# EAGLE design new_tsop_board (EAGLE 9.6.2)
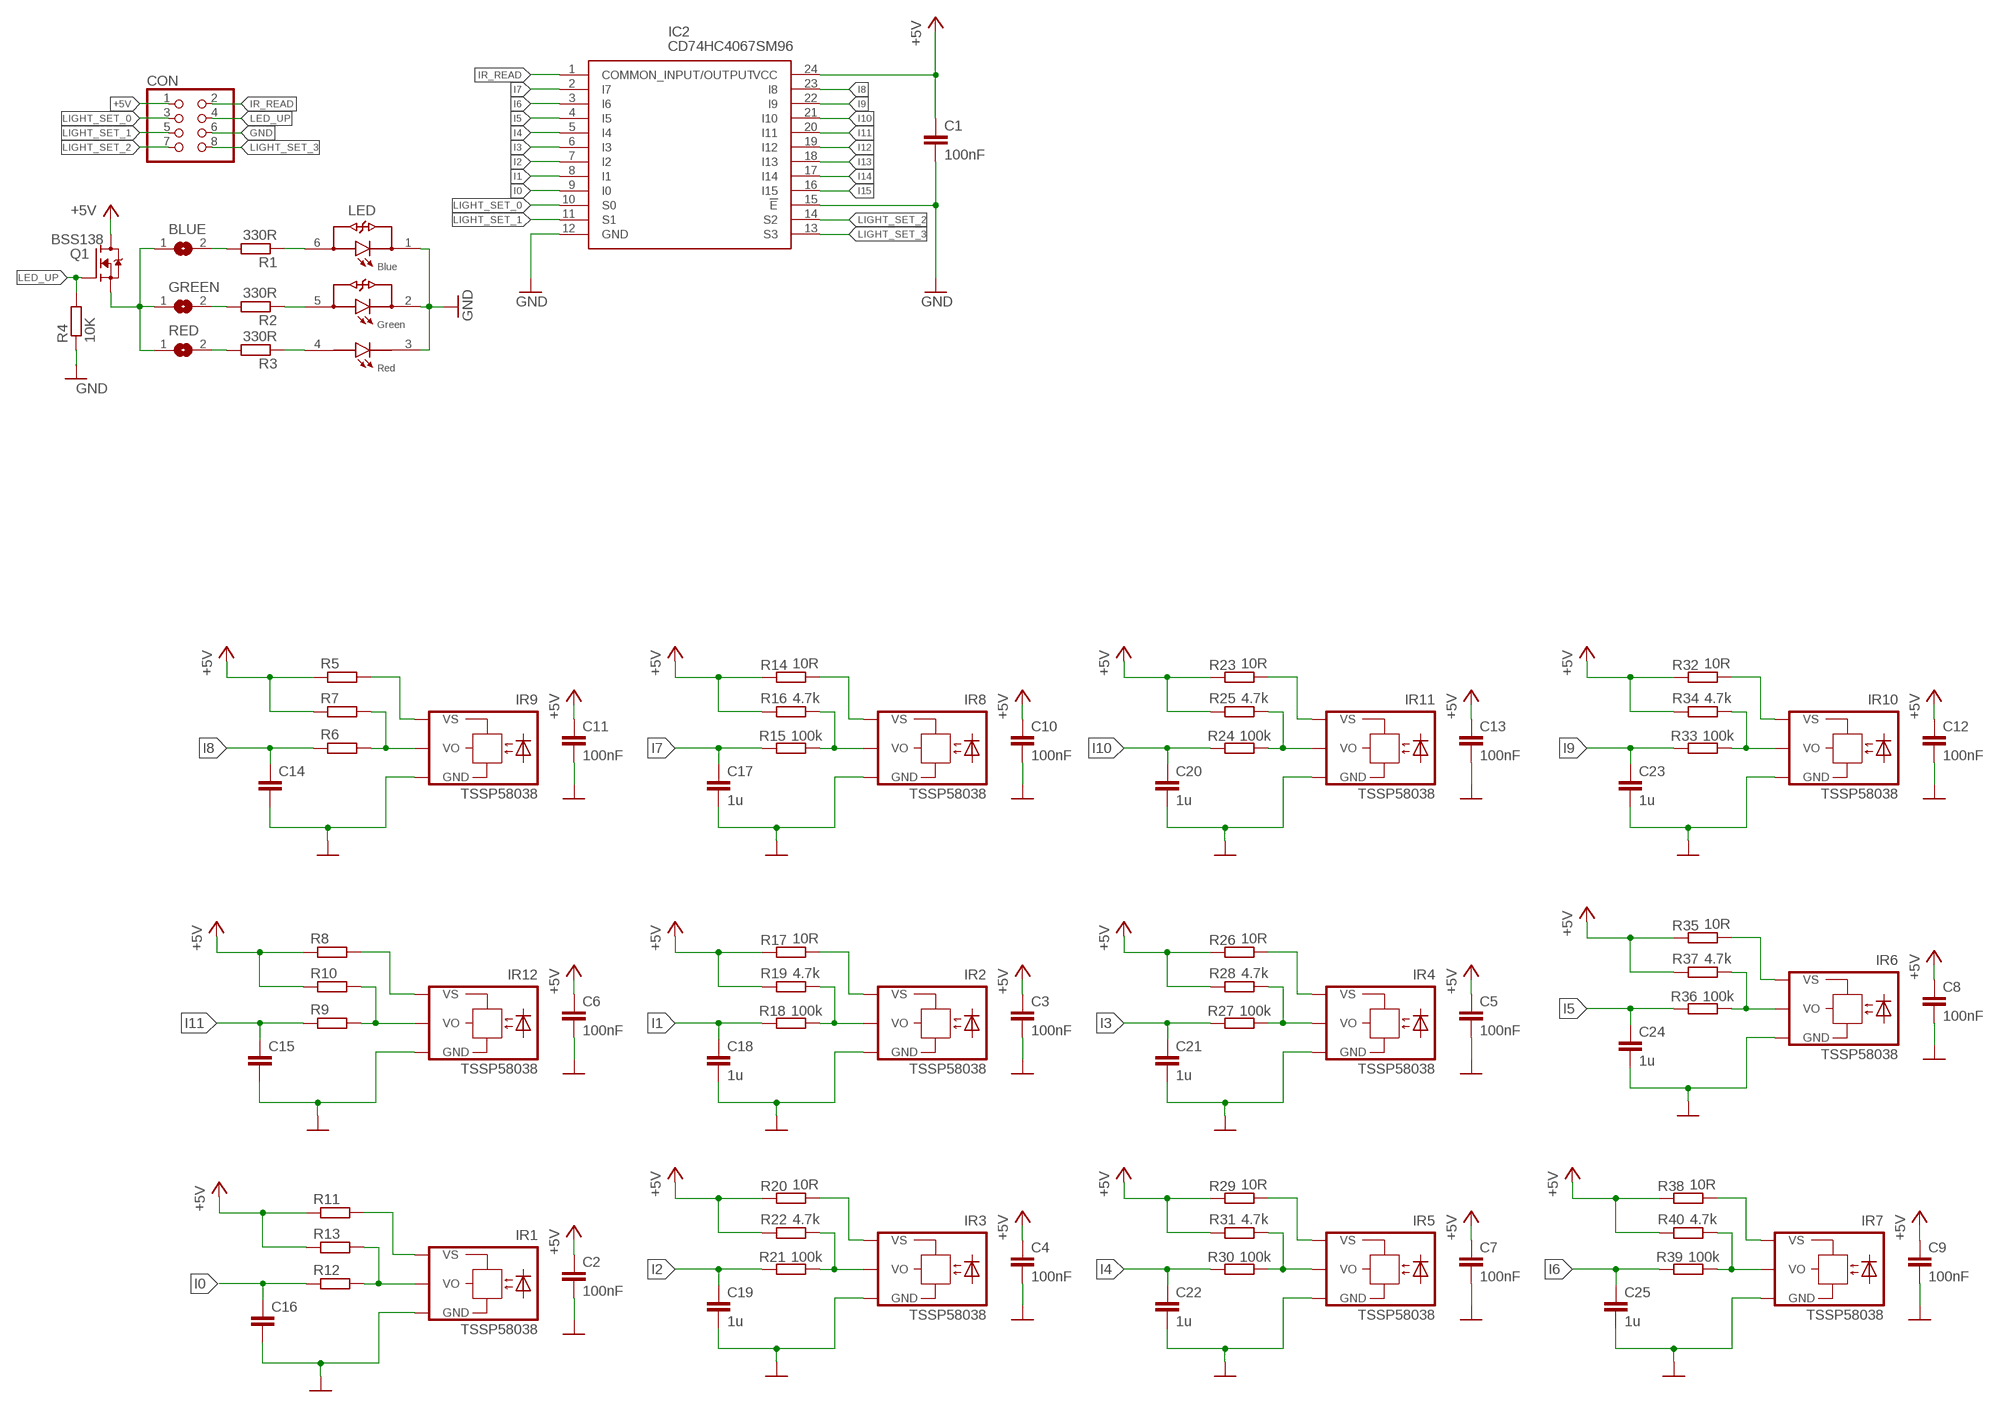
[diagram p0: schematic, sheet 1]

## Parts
BLUE  SJ  [SJ]
C1  100nF  C-EUC0805  [C0805]
C2  100nF  C-EUC0805  [C0805]
C3  100nF  C-EUC0805  [C0805]
C4  100nF  C-EUC0805  [C0805]
C5  100nF  C-EUC0805  [C0805]
C6  100nF  C-EUC0805  [C0805]
C7  100nF  C-EUC0805  [C0805]
C8  100nF  C-EUC0805  [C0805]
C9  100nF  C-EUC0805  [C0805]
C10  100nF  C-EUC0805  [C0805]
C11  100nF  C-EUC0805  [C0805]
C12  100nF  C-EUC0805  [C0805]
C13  100nF  C-EUC0805  [C0805]
C14  C-EUC0805  [C0805]
C15  C-EUC0805  [C0805]
C16  C-EUC0805  [C0805]
C17  1u  C-EUC0805  [C0805]
C18  1u  C-EUC0805  [C0805]
C19  1u  C-EUC0805  [C0805]
C20  1u  C-EUC0805  [C0805]
C21  1u  C-EUC0805  [C0805]
C22  1u  C-EUC0805  [C0805]
C23  1u  C-EUC0805  [C0805]
C24  1u  C-EUC0805  [C0805]
C25  1u  C-EUC0805  [C0805]
CON  PINHD-2X4  [2X04]
GREEN  SJ  [SJ]
IC2  CD74HC4067SM96  [SOP65P780X200-24N]
IR1  TSSP58038  TSOP4038  [TSOP]
IR2  TSSP58038  TSOP4038  [TSOP]
IR3  TSSP58038  TSOP4038  [TSOP]
IR4  TSSP58038  TSOP4038  [TSOP]
IR5  TSSP58038  TSOP4038  [TSOP]
IR6  TSSP58038  TSOP4038  [TSOP]
IR7  TSSP58038  TSOP4038  [TSOP]
IR8  TSSP58038  TSOP4038  [TSOP]
IR9  TSSP58038  TSOP4038  [TSOP]
IR10  TSSP58038  TSOP4038  [TSOP]
IR11  TSSP58038  TSOP4038  [TSOP]
IR12  TSSP58038  TSOP4038  [TSOP]
LED  LTST-G563ZEGBW  [LED_LTST-G563ZEGBW]
Q1  BSS138  [SOT95P240X111-3N]
R1  330R  R-EU_R1206  [R1206]
R2  330R  R-EU_R1206  [R1206]
R3  330R  R-EU_R1206  [R1206]
R4  10K  R-EU_R1206  [R1206]
R5  R-EU_R0805  [R0805]
R6  R-EU_R0805  [R0805]
R7  R-EU_R0805  [R0805]
R8  R-EU_R0805  [R0805]
R9  R-EU_R0805  [R0805]
R10  R-EU_R0805  [R0805]
R11  R-EU_R0805  [R0805]
R12  R-EU_R0805  [R0805]
R13  R-EU_R0805  [R0805]
R14  10R  R-EU_R0805  [R0805]
R15  100k  R-EU_R0805  [R0805]
R16  4.7k  R-EU_R0805  [R0805]
R17  10R  R-EU_R0805  [R0805]
R18  100k  R-EU_R0805  [R0805]
R19  4.7k  R-EU_R0805  [R0805]
R20  10R  R-EU_R0805  [R0805]
R21  100k  R-EU_R0805  [R0805]
R22  4.7k  R-EU_R0805  [R0805]
R23  10R  R-EU_R0805  [R0805]
R24  100k  R-EU_R0805  [R0805]
R25  4.7k  R-EU_R0805  [R0805]
R26  10R  R-EU_R0805  [R0805]
R27  100k  R-EU_R0805  [R0805]
R28  4.7k  R-EU_R0805  [R0805]
R29  10R  R-EU_R0805  [R0805]
R30  100k  R-EU_R0805  [R0805]
R31  4.7k  R-EU_R0805  [R0805]
R32  10R  R-EU_R0805  [R0805]
R33  100k  R-EU_R0805  [R0805]
R34  4.7k  R-EU_R0805  [R0805]
R35  10R  R-EU_R0805  [R0805]
R36  100k  R-EU_R0805  [R0805]
R37  4.7k  R-EU_R0805  [R0805]
R38  10R  R-EU_R0805  [R0805]
R39  100k  R-EU_R0805  [R0805]
R40  4.7k  R-EU_R0805  [R0805]
RED  SJ  [SJ]

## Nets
+5V: C1.1 C2.1 C3.1 C4.1 C5.1 C6.1 C7.1 C8.1 C9.1 C10.1 C11.1 C12.1 C13.1 CON.1 IC2.24(VCC) Q1.3(D) R5.1 R7.1 R8.1 R10.1 R11.1 R13.1 R14.1 R16.1 R17.1 R19.1 R20.1 R22.1 R23.1 R25.1 R26.1 R28.1 R29.1 R31.1 R32.1 R34.1 R35.1 R37.1 R38.1 R40.1
GND: C1.2 C2.2 C3.2 C4.2 C5.2 C6.2 C7.2 C8.2 C9.2 C10.2 C11.2 C12.2 C13.2 C14.2 C15.2 C16.2 C17.2 C18.2 C19.2 C20.2 C21.2 C22.2 C23.2 C24.2 C25.2 CON.6 IC2.12(GND) IC2.15(!E) IR1.GND IR2.GND IR3.GND IR4.GND IR5.GND IR6.GND IR7.GND IR8.GND IR9.GND IR10.GND IR11.GND IR12.GND LED.1 LED.2 LED.3 R4.1
I0: C16.1 IC2.9(I0) R12.1
I1: C18.1 IC2.8(I1) R18.1
I2: C19.1 IC2.7(I2) R21.1
I3: C21.1 IC2.6(I3) R27.1
I4: C22.1 IC2.5(I4) R30.1
I5: C24.1 IC2.4(I5) R36.1
I6: C25.1 IC2.3(I6) R39.1
I7: C17.1 IC2.2(I7) R15.1
I8: C14.1 IC2.23(I8) R6.1
I9: C23.1 IC2.22(I9) R33.1
I10: C20.1 IC2.21(I10) R24.1
I11: C15.1 IC2.20(I11) R9.1
I12: IC2.19(I12)
I13: IC2.18(I13)
I14: IC2.17(I14)
I15: IC2.16(I15)
IR_READ: CON.2 IC2.1(COMMON_INPUT/OUTPUT)
LED_UP: CON.4 Q1.1(G) R4.2
LIGHT_SET_0: CON.3 IC2.10(S0)
LIGHT_SET_1: CON.5 IC2.11(S1)
LIGHT_SET_2: CON.7 IC2.14(S2)
LIGHT_SET_3: CON.8 IC2.13(S3)
N$1: LED.6 R1.1
N$2: LED.5 R2.1
N$3: LED.4 R3.1
N$4: R3.2 RED.2
N$5: GREEN.2 R2.2
N$6: BLUE.2 R1.2
N$7: BLUE.1 GREEN.1 Q1.2(S) RED.1
N$8: IR12.VS R8.2
N$9: IR1.VS R11.2
N$10: IR8.VS R14.2
N$11: IR2.VS R17.2
N$12: IR3.VS R20.2
N$13: IR11.VS R23.2
N$14: IR4.VS R26.2
N$15: IR5.VS R29.2
N$16: IR10.VS R32.2
N$17: IR9.VS R5.2
N$18: IR6.VS R35.2
N$19: IR7.VS R38.2
N$20: IR12.VO R9.2 R10.2
N$21: IR9.VO R6.2 R7.2
N$22: IR5.VO R30.2 R31.2
N$23: IR1.VO R12.2 R13.2
N$25: IR8.VO R15.2 R16.2
N$26: IR4.VO R27.2 R28.2
N$27: IR2.VO R18.2 R19.2
N$29: IR11.VO R24.2 R25.2
N$30: IR3.VO R21.2 R22.2
N$32: IR10.VO R33.2 R34.2
N$34: IR6.VO R36.2 R37.2
N$36: IR7.VO R39.2 R40.2

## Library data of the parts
BLUE GREEN RED = jumper:SJ: SMD solder JUMPER
C1-C25 = rcl:C-EU: CAPACITOR, European symbol; SPICEPREFIX: C
CON = pinhead:PINHD-2X4: PIN HEADER
IC2 = SamacSys_Parts:CD74HC4067SM96: High Speed CMOS 16-Ch MUX/DEMUX 24P SOIC CD74HC4067SM96, Multiplexer/Demultiplexer Single 16:1, 3 V, 5 V, 24-Pin, SSOP, 1 Source: Datasheet; DESCRIPTION: High Speed CMOS 16-Ch MUX/DEMUX 24P SOIC CD74HC4067SM96, Multiplexer/Demultiplexer Single 16:1, 3 V, 5 V, 24-Pin, SSOP, 1; HEIGHT: 2mm; MANUFACTURER_NAME: Texas Instruments; MANUFACTURER_PART_NUMBER: CD74HC4067SM96; MOUSER_PART_NUMBER: 595-CD74HC4067SM96; MOUSER_PRICE-STOCK: https://www.mouser.co.uk/ProductDetail/Texas-Instruments/CD74HC4067SM96?qs=JHHQeKcAU3DyfvAOSRLjhQ%3D%3D
IR1-IR12 = TSOP4038:TSOP4038: TSOP4038 IR Receiver Module Source: http://www.vishay.com/docs/81926/tsop4038.pdf Check availability; AVAILABILITY: In Stock; DESCRIPTION: Remote Receiver Sensor, 38.0kHz 30m Through Hole; MF: Vishay; MP: TSOP4038; PACKAGE: None; PRICE: None; PURCHASE-URL: https://pricing.snapeda.com/search/part/TSOP4038/?ref=eda
LED = LTST-G563ZEGBW:LTST-G563ZEGBW: LED; SMD; 5050, PLCC6; RGB; 5x5x1.6mm; 120°; 20mA; Lens: transparent Check availability; AVAILABILITY: Not in stock; DESCRIPTION: LED; SMD; 5050, PLCC6; RGB; 5x5x1.6mm; 120°; 20mA; Lens: transparent; MF: Lite-On; MP: LTST-G563ZEGBW; PACKAGE: PLCC-6 Lite-On; PRICE: None
Q1 = BSS138:BSS138: N-Channel 50V 220mA (Ta) 360mW (Ta) Surface Mount SOT-23-3 Check availability; AVAILABILITY: In Stock; DESCRIPTION: N-Channel 50 V 200mA (Ta) 225mW (Ta) Surface Mount SOT-23-3 (TO-236); MF: ON Semiconductor; MP: BSS138; PACKAGE: SOT-23 ON; PRICE: None; PURCHASE-URL: https://pricing.snapeda.com/search/part/BSS138/?ref=eda
R1-R40 = rcl:R-EU_: RESISTOR, European symbol; SPICEPREFIX: R

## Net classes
0 default: clearance 0.205 mm

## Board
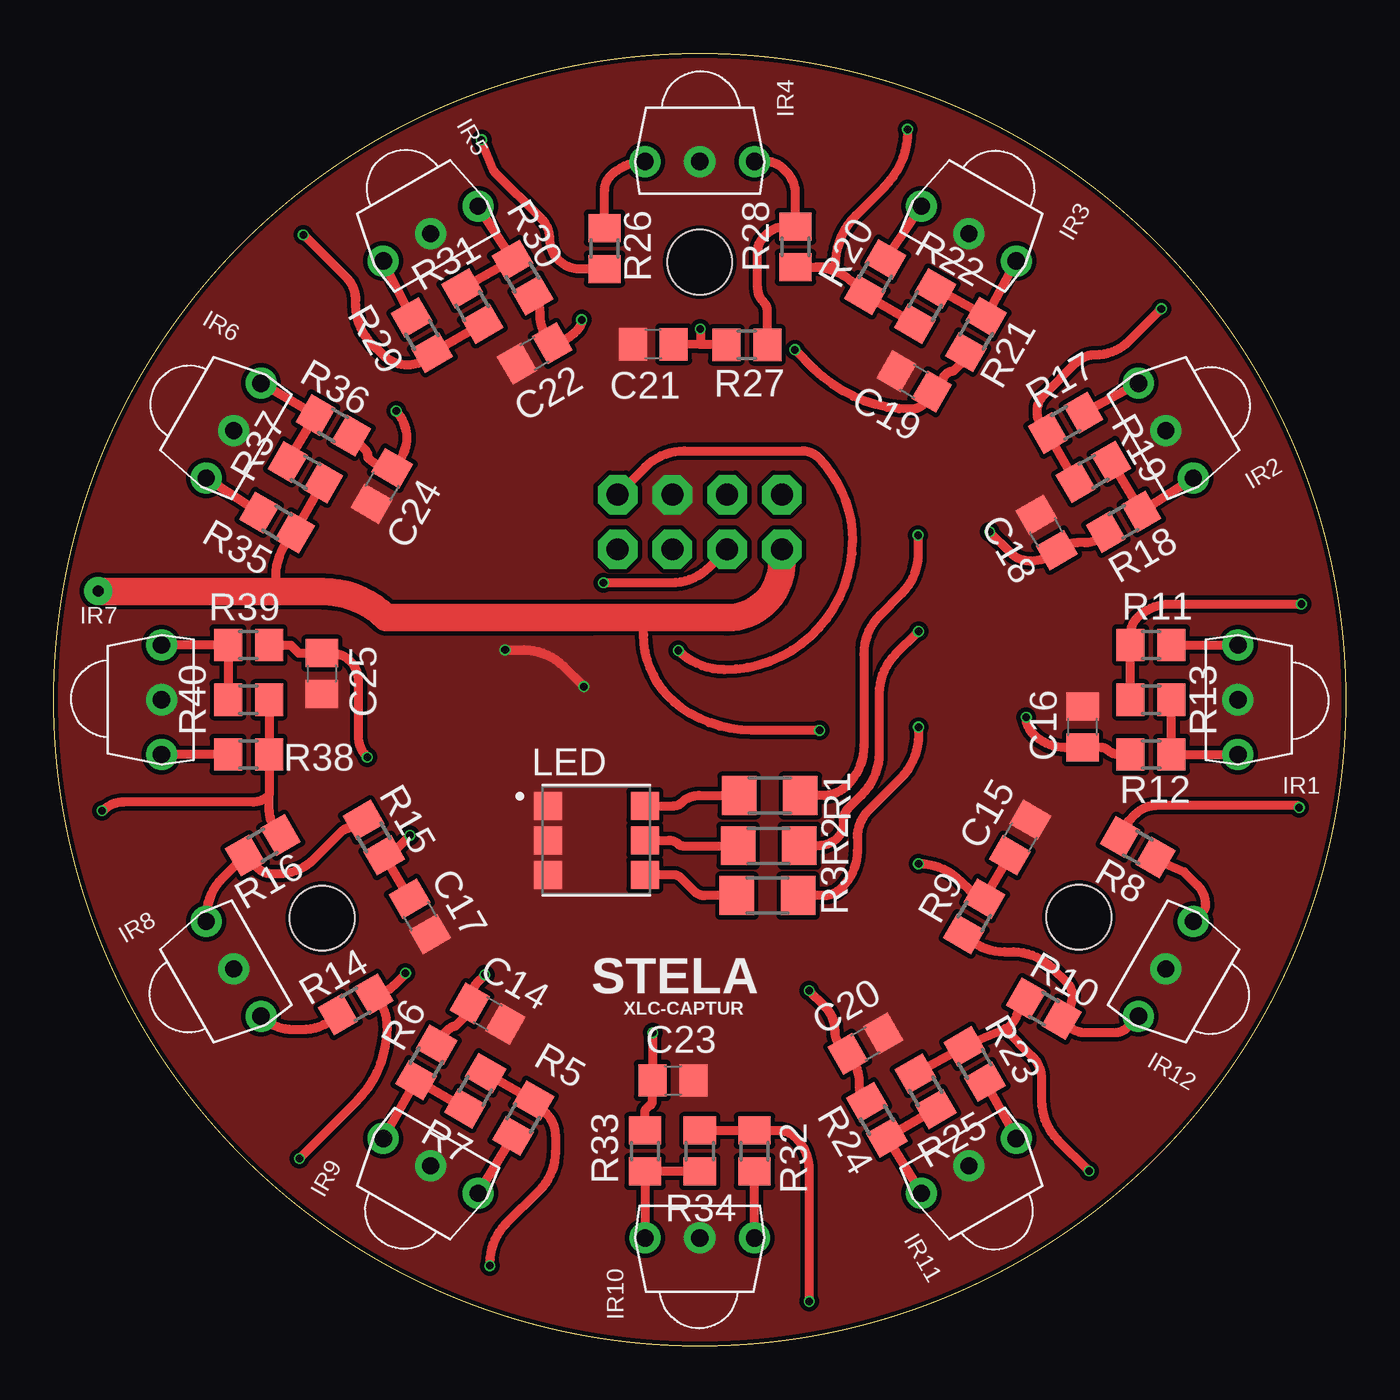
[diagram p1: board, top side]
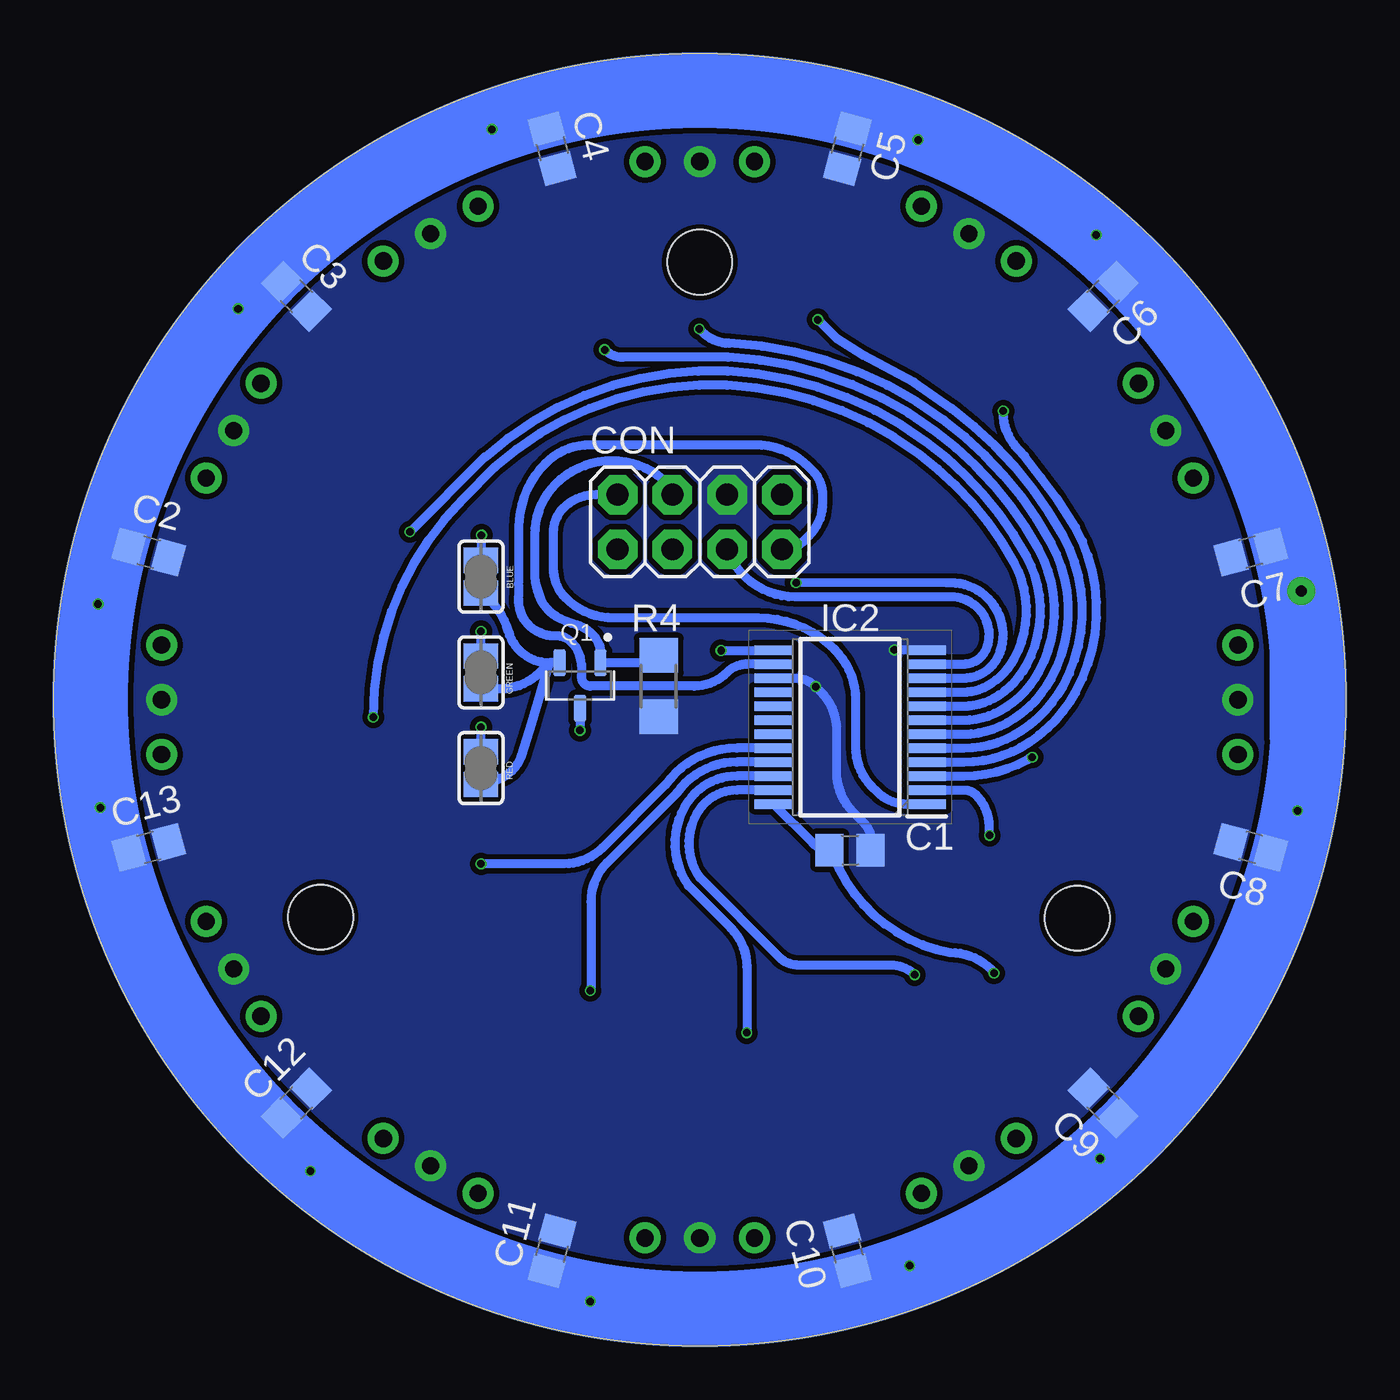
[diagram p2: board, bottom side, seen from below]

Size 60 x 60 mm. Coordinates in mm from the lower left corner, seen from the top.
Outline: circle at 30,30 radius 30
Copper layers (1*16): Top 0.035mm / dielectric 1.6mm / Bottom 0.035mm
Design rules "jlc_pcb": minimum track width 5mil, minimum drill 0.3mm, track to track 5mil, track to pad 5mil, pad to pad 5mil, via to via 5mil, smd to smd 5mil, copper to edge 0.2mm, drill to drill 6mil, minimum pad ring 10mil, minimum via ring 3mil, stop-mask expansion 4mil, vias tented up to drill 0mil, thermal gap 10mil
Holes 3 mm at 30,50.32 47.61,19.9 12.46,19.86

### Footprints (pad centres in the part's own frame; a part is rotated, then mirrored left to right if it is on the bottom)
SJ = smd 1.168 x 1.6: 1 -0.762,0; 2 0.762,0
C0805 = smd 1.3 x 1.5: 1 -0.95,0; 2 0.95,0
2X04 = drill 1.016 octagon: 1 -3.81,-1.27; 2 -3.81,1.27; 3 -1.27,-1.27; 4 -1.27,1.27; 5 1.27,-1.27; 6 1.27,1.27; 7 3.81,-1.27; 8 3.81,1.27
SOP65P780X200-24N = smd 1.8 x 0.45: 1 -3.55,3.575; 2 -3.55,2.925; 3 -3.55,2.275; 4 -3.55,1.625; 5 -3.55,0.975; 6 -3.55,0.325; 7 -3.55,-0.325; 8 -3.55,-0.975; 9 -3.55,-1.625; 10 -3.55,-2.275; 11 -3.55,-2.925; 12 -3.55,-3.575; 13 3.55,-3.575; 14 3.55,-2.925; 15 3.55,-2.275; 16 3.55,-1.625; 17 3.55,-0.975; 18 3.55,-0.325; 19 3.55,0.325; 20 3.55,0.975; 21 3.55,1.625; 22 3.55,2.275; 23 3.55,2.925; 24 3.55,3.575
TSOP = drill 0.8: GND 0,0; VO 0,-2.54; VS 0,2.54
LED_LTST-G563ZEGBW = smd 1.3 x 1.3: 1 -2.25,1.6; 2 -2.25,0; 3 -2.25,-1.6; 4 2.25,-1.6; 5 2.25,0; 6 2.25,1.6
SOT95P240X111-3N = smd 1.23 x 0.6: 1 -1.06,0.95; 2 -1.06,-0.95; 3 1.06,0
R1206 = smd 1.6 x 1.803: 1 -1.422,0; 2 1.422,0
R0805 = smd 1.3 x 1.5: 1 -0.95,0; 2 0.95,0

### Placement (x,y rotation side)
BLUE  40.16,35.72 90 bottom
C1  23.02,23.02 0 bottom
C2  55.6,36.86 345 bottom
C3  48.74,48.74 315 bottom
C4  36.86,55.6 285 bottom
C5  23.14,55.6 255 bottom
C6  11.26,48.74 225 bottom
C7  4.4,36.86 195 bottom
C8  4.4,23.14 165 bottom
C9  11.26,11.26 135 bottom
C10  23.14,4.4 105 bottom
C11  36.86,4.4 75 bottom
C12  48.74,11.26 45 bottom
C13  55.6,23.14 15 bottom
C14  20.14,15.42 330 top
C15  44.88,23.6 60 top
C16  47.78,28.73 90 top
C17  17,19.94 300 top
C18  46.1,37.77 120 top
C19  39.96,44.78 150 top
C20  37.7,14.02 30 top
C21  27.84,46.51 180 top
C22  22.33,46.08 210 top
C23  28.76,12.32 0 top
C24  15.24,39.93 240 top
C25  12.45,31.22 270 top
CON  30,38.26 0 bottom
GREEN  40.16,31.27 90 bottom
IC2  23.02,28.73 180 bottom
IR1  55,30 0 top
IR2  51.65,42.5 30 top
IR3  42.5,51.65 60 top
IR4  30,55 90 top
IR5  17.5,51.65 120 top
IR6  8.35,42.5 150 top
IR7  5,30 180 top
IR8  8.35,17.5 210 top
IR9  17.5,8.35 240 top
IR10  30,5 270 top
IR11  42.5,8.35 300 top
IR12  51.65,17.5 330 top
LED  25.2,23.47 0 top
Q1  35.56,30.66 270 bottom
R1  33.25,25.55 0 top
R2  33.2,23.22 0 top
R3  33.15,20.91 0 top
R4  31.91,30.64 90 bottom
R5  21.8,10.57 240 top
R6  17.3,13.16 240 top
R7  19.59,11.84 240 top
R8  50.35,23.14 330 top
R9  42.75,19.94 240 top
R10  45.98,15.65 330 top
R11  50.95,32.54 0 top
R12  50.95,27.46 0 top
R13  50.95,30 0 top
R14  14.02,15.85 210 top
R15  14.86,23.6 120 top
R16  9.71,23.24 210 top
R17  46.99,42.85 30 top
R18  49.69,38.26 30 top
R19  48.29,40.59 30 top
R20  38.15,49.63 60 top
R21  42.83,46.97 60 top
R22  40.46,48.29 60 top
R23  42.78,13.08 300 top
R24  38.23,10.49 300 top
R25  40.49,11.81 300 top
R26  25.58,50.95 90 top
R27  32.18,46.48 0 top
R28  34.45,51.03 90 top
R29  17.1,46.94 120 top
R30  21.77,49.61 120 top
R31  19.43,48.29 120 top
R32  32.54,9.05 270 top
R33  27.46,9.05 270 top
R34  30,9.05 270 top
R35  10.37,38.23 150 top
R36  12.98,42.75 150 top
R37  11.69,40.57 150 top
R38  9.05,27.46 180 top
R39  9.05,32.54 180 top
R40  9.05,30 180 top
RED  40.16,26.82 90 bottom

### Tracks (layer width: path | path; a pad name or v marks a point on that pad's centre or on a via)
+5V  (via drill 0.35, 0.5 pad 1.3)
  Top 0.406: v35.56,28.58 32.42,28.58 arc-36 29.13,29.64 arc-65 27.46,33.81 | R13.1 R11.1 50,33.05 arc-45 50.32,33.81 arc-45 51.85,34.45 v57.94,34.45 | R34.1 R32.1 33.69,10 arc-45 34.45,9.68 arc-45 35.08,8.15 v35.08,2.06 | R25.1 42.21,13.86 42.25,13.88 | 42.25,13.88 42.55,14.04 44.16,14.71 | 42.25,13.88 R23.1 | R19.1 R17.1 46.05,42.5 arc-45 45.67,43.41 arc-45 45.98,44.15 47.48,45.65 arc-45 48.39,46.03 arc45 49.95,46.67 v51.44,48.16 | R31.1 R29.1 17.39,45.94 arc-45 16.44,45.55 arc-45 15.27,46.03 14.77,46.53 arc-45 14.02,48.32 14.02,48.57 arc45 13.59,49.61 11.63,51.57 arc45 v11.59,51.59 | R37.1 R35.1 11.14,37.7 arc45 10.32,35.72 10.32,35.03 | R40.1 R38.1 10,25.55 | R7.1 R5.1 22.86,10.8 arc-45 23.29,9.76 23.29,9 arc-45 22.55,7.21 20.99,5.65 arc45 20.25,3.85 v20.25,3.71 | R10.1 44.81,15.78 arc-45 44.43,14.88 44.34,14.79 arc-45 44.16,14.71 | 34.79,50.08 R28.1 35.36,50.08 | R16.1 arc-45 10,25.01 10,25.55 | 44.16,14.71 45.44,13.44 arc-45 45.88,12.38 45.88,11.37 arc45 46.62,9.57 v48.09,8.11 | R8.1 49.66,23.75 arc45 49.91,24.35 50.26,24.71 arc-45 51.2,25.1 57.74,25.1 v57.84,25 | v39.65,56.49 39.65,56.45 arc-45 38.55,53.79 37.25,52.49 arc45 36.28,50.15 arc-45 36.12,50.08 35.36,50.08 | 35.36,50.08 arc-45 37.15,49.34 R20.1 R22.1 | v19.87,56.01 arc45 19.87,55.95 20.45,54.54 22.64,52.34 arc-45 23.04,51.39 arc45 23.44,50.43 23.48,50.39 | R26.1 24.41,50 arc-45 23.48,50.39 | 23.48,50.39 | 10,25.55 arc-45 9.26,25.25 3.23,25.25 arc45 2.31,24.87 arc-45 2.25,24.84 v2.24,24.84 | v11.41,8.69 14.01,11.3 arc45 15.47,14.82 arc45 R14.1 arc45 15.77,16.71 16.34,17.27 v16.34,17.3
  Top 1.27: CON.1 33.81,36.35 arc-90 31.27,33.81 27.46,33.81 24.92,33.81 | 24.92,33.81 24.45,33.81 | v2.06,35.05 2.09,35.03 10.32,35.03 12.49,35.03 arc-45 15.44,33.81 24.92,33.81
  Bottom 0.127: C8.1 3.16,24.99 2.77,27.46 3.48,28.17 3.48,35.08 C7.1 3.48,40.16 4.71,41.39 4.71,43.53 C6.1 12.18,51 14.04,52.86 14.12,52.86 17.27,56.01 v19.87,56.01 22.39,56.01 C5.1 24.24,57.86 35.76,57.86 C4.1 37.74,57.15 39.61,57.15 39.8,56.95 41.79,54.97 43.86,54.97 C3.1 51.05,47.77 52.75,46.08 52.75,45.84 56.67,41.91 56.67,36.35 56.52,36.51 C2.1 57.23,36.39 57.23,34.45 57.23,24.92 57.23,23.61 C13.1 56.52,20.48 54.65,18.61 54.65,15.83 C12.1 49.41,10.2 47.7,8.49 42.7,3.48 C11.1 36.39,2.77 35.08,2.77 23.61,2.77 C10.1 20.48,3.48 v20.25,3.71 18.61,5.35 15.83,5.35 12.18,9 C9.1 7.89,13.29 7.89,14.16
  Bottom 0.254: 3.48,35.08 arc-45 3.42,35.05 v2.06,35.05
  Bottom 0.406: IC2.24 24.75,23.34 arc-45 C1.1 23.53,22.14 arc-53 18.36,18.26 arc45 16.46,17.47 16.37,17.39 arc45 v16.34,17.3 | Q1.3 v35.56,28.58 | v35.08,2.06 35.08,2.77 | v48.09,8.11 47.7,8.49 | v57.84,25 arc-45 57.65,24.92 57.23,24.92 | v57.94,34.45 57.23,34.45 | v51.44,48.16 51.05,47.77 | 51.05,47.77 arc45 51.05,47.77 | 39.8,56.95 arc-45 39.61,56.47 arc-45 v39.65,56.49 | v11.59,51.59 12.18,51 | 12.18,51 arc45 12.18,51 | v2.24,24.84 2.8,24.84 arc45 3.16,24.99 | v11.41,8.69 arc-45 12.16,9 12.18,9
  Bottom 1.27: 42.02,55.28 41.79,54.97
GND  (via drill 0.35)
  Top 0.406: v20.96,32.31 21.86,32.31 arc-45 23.66,31.57 v24.62,30.61
  Bottom 0.406: IC2.15 25.57,31 arc45 v24.62,30.61 24.39,30.39 arc45 23.65,28.59 23.65,26.61 arc-45 22.91,24.81 22.38,24.29 arc45 22.07,23.52 C1.2 | IC2.12 20.94,32.3 arc45 v20.96,32.31
  pour Top (no thermals): -1.11,-1.11 -1.11,61.11 61.11,61.11 61.11,-1.11
  pour Bottom (isolate 0.254, no thermals): -1.11,61.11 61.11,61.11 61.11,-1.11 -1.11,-1.11
I0  (via drill 0.35)
  Top 0.406: R12.1 49.44,27.46 arc-45 48.95,27.66 arc45 48.67,27.78 C16.1 | C16.1 47.64,27.64 | C16.1 46.98,27.78 arc-45 45.5,28.4 45.49,28.41 arc-45 v45.16,29.19
  Bottom 0.406: IC2.9 17.75,30.36 arc-29 16.66,30.64 arc-32 15.39,31.91 arc-58 15.39,36.35 arc-25 19.84,41.43 arc-34 28.73,44.61 arc-44 39.52,40.8 40.99,39.33 arc-45 45.18,29.22 arc45 v45.16,29.19
I1  (via drill 0.35)
  Top 0.406: 48.78,37.69 R18.1 48.7,37.62 arc-45 47.91,37.29 47.53,37.29 arc45 46.71,36.95 | 46.98,36.95 46.71,36.95 | 46.71,36.95 C18.1 arc-45 45.38,36.45 45.34,36.45 arc-45 44.43,36.83 v43.46,37.8
  Bottom 0.406: IC2.8 17.75,29.7 arc-29 16.35,30.07 arc-32 14.83,31.59 arc-58 14.83,36.66 arc-25 19.45,41.95 arc-34 28.7,45.25 arc-44 39.96,41.28 arc-45 39.99,41.27 v43.46,37.8
I2  (via drill 0.35)
  Top 0.406: R21.1 arc-45 42.13,45.61 41.79,45.27 arc45 41.44,45.12 41.33,45.01 arc-45 41.22,44.75 C19.1 arc-45 40.64,43.97 40.41,43.74 arc-45 39.82,43.49 arc-45 35.31,45.36 v34.42,46.26
  Bottom 0.406: IC2.7 17.75,29.05 arc-29 16.04,29.5 arc-32 14.26,31.28 arc-58 14.26,36.98 arc-25 19.07,42.48 arc-34 28.67,45.9 33.57,45.9 arc45 v34.42,46.26
I3  (via drill 0.35)
  Top 0.406: R27.1 30,46.5 | 30,46.5 C21.1 | v30.02,47.22 30.02,46.56 arc-45 30,46.5
  Bottom 0.406: IC2.6 17.75,28.41 arc-29 15.72,28.93 arc-32 13.69,30.96 arc-58 13.69,37.29 arc-25 18.68,43 arc-34 28.64,46.55 arc45 29.87,47.06 v30.02,47.22
I4  (via drill 0.35)
  Top 0.406: C22.1 23.12,46.59 | 23.12,46.59 arc-45 22.58,47.88 22.58,47.97 arc45 R30.1 | v24.51,47.65 arc-45 24.32,47.18 24.16,47.02 arc-45 23.12,46.59
  Bottom 0.406: IC2.5 17.75,27.75 arc-29 15.41,28.36 arc-32 13.12,30.65 arc-58 13.12,37.61 arc-25 18.29,43.52 arc45 18.3,43.52 20.07,44.76 22.41,45.99 23.62,46.76 v24.51,47.65
I5  (via drill 0.35)
  Top 0.406: R36.1 14.42,41.66 arc-45 14.59,41.24 14.63,41.2 arc45 C24.1 15.89,40.93 arc45 16.41,42.17 arc45 15.9,43.38 v15.9,43.41
  Bottom 0.406: IC2.4 17.75,27.11 arc-29 15.1,27.79 arc-32 12.55,30.34 arc-58 12.55,38.01 | 12.55,38.01 | 12.55,38.01 13.41,39.35 14.15,40.31 14.91,41.33 15.16,41.58 arc45 15.9,43.37 v15.9,43.41
I6  (via drill 0.35)
  Top 0.406: R39.1 10.95,32.54 arc-45 11.04,32.5 11.36,32.18 arc45 11.39,32.17 C25.1 12.47,32.14 12.93,32.14 arc-45 13.77,31.8 arc-45 14.15,30.87 14.15,28.31 arc45 v14.56,27.33
  Bottom 0.406: IC2.3 17.75,26.45 arc-29 14.78,27.22 arc45 14.54,27.32 v14.56,27.33
I7  (via drill 0.35)
  Top 0.406: C17.1 R15.1 arc45 15.61,22.78 v16.54,23.7
  Bottom 0.406: IC2.2 17.94,25.8 | 17.94,25.8 17.75,25.8 | 17.94,25.8 17.71,25.8 arc45 17.17,25.58 arc45 16.56,24.11 16.56,23.76 arc45 v16.54,23.7
I8  (via drill 0.35)
  Top 0.406: R6.1 arc-45 17.87,14.21 18.39,14.73 arc-45 18.65,14.84 19.05,15.24 arc45 C14.1 arc-45 19.77,16.98 v20.02,17.22
  Bottom 0.406: IC2.23 28.28,25.8 arc-54 30,24.92 arc-71 30,21.74 26.3,18.04 arc-45 25.42,17.68 21.12,17.68 arc45 v20.02,17.22
I9  (via drill 0.35)
  Top 0.406: R33.1 27.46,10.95 27.67,11.16 arc-45 27.71,11.18 arc45 27.8,11.4 C23.1 arc45 27.82,12.35 v27.82,14.53
  Bottom 0.406: IC2.22 28.28,26.45 arc-54 30.53,25.3 arc-71 30.53,21.37 28.56,19.4 arc45 27.82,17.6 v27.82,14.53
I10  (via drill 0.35)
  Top 0.406: R24.1 37.69,11.38 arc-45 37.42,12.04 37.42,12.24 arc45 C20.1 36.6,13.82 arc-45 36.27,14.61 arc45 35.79,15.78 v35.08,16.49
  Bottom 0.406: IC2.21 28.28,27.11 arc-54 31.06,25.68 34.31,22.42 arc-45 35.05,20.63 35.05,16.49 v35.08,16.49
I11  (via drill 0.35)
  Top 0.406: C15.1 R9.1 43.07,20.92 arc-45 42.55,21.14 42.11,21.57 arc45 v40.16,22.38
  Bottom 0.406: IC2.20 28.28,27.75 arc-54 31.59,26.05 34.52,23.12 arc45 36.31,22.38 v40.16,22.38
IR_READ
  Bottom 0.406: IC2.1 20.38,25.16 arc45 21.77,25.73 22.02,25.98 arc45 22.76,27.78 22.76,29.96 arc-45 23.75,32.35 arc-45 27.27,33.81 34,33.81 arc45 36.24,34.74 arc45 36.81,36.1 36.81,37.79 arc45 36.35,38.89 arc45 34.82,39.52 CON.2
LED_UP
  Bottom 0.406: CON.4 arc-45 31.47,40.02 arc-45 34.08,41.1 arc-45 36.7,40.01 arc-45 37.67,37.68 37.67,35.92 arc-25 37.39,34.66 arc-34 36.69,33.9 arc-15 35.7,33.47 arc85 Q1.1 31.91,31.72 R4.2
LIGHT_SET_0  (via drill 0.35)
  Top 0.406: v25.53,35.44 28.67,35.44 arc45 30.46,36.18 CON.3
  Bottom 0.406: IC2.10 17.75,31 arc-70 16.05,32.19 arc-75 16.93,34.98 arc-39 18.54,35.42 v25.53,35.44
LIGHT_SET_1
  Bottom 0.406: IC2.11 17.75,31.66 arc-70 16.66,32.41 arc-75 17.3,34.45 arc-39 18.49,34.77 25.55,34.77 arc70 CON.5
LIGHT_SET_2
  Bottom 0.406: CON.7 arc-45 25.11,37.43 24.92,37.62 arc-45 24.29,39.15 24.29,39.52 arc-45 24.73,40.61 24.92,40.8 arc-45 27.43,41.84 35.09,41.84 arc-45 37.17,40.98 arc-45 38.41,37.99 38.41,35.47 arc4 38.41,34.67 arc-40 38.07,33.61 arc-56 36.66,32.97 arc31 36.25,32.88 arc42 35.61,32.16 arc27 35.49,31.09 arc-97 35.08,30.64 30.26,30.64 arc-45 28.73,31.27 arc45 27.8,31.66 IC2.14
LIGHT_SET_3  (via drill 0.35)
  Top 0.406: CON.8 27.48,40.81 arc-45 29.27,41.56 34.79,41.56 arc-45 35.48,41.27 arc-45 37.1,37.36 arc-90 31.14,31.4 arc-45 v29.01,32.29
  Bottom 0.406: v29.01,32.29 26.61,32.29 arc-45 IC2.13
N$1
  Top 0.406: LED.6 28.79,25.07 arc45 29.16,25.23 arc-45 29.96,25.55 R1.1
N$2
  Top 0.406: LED.5 28.58,23.47 arc-45 29.01,23.29 arc45 29.19,23.22 R2.1
N$3
  Top 0.406: R3.1 30.2,20.91 arc-45 29.77,21.09 29.15,21.71 arc45 28.75,21.87 LED.4 arc-45 LED.4
N$4  (via drill 0.35)
  Top 0.406: v40.16,28.73 40.16,28.39 arc-45 39.31,26.33 37.82,24.84 arc45 37.31,23.62 37.31,22.98 arc-45 36.62,21.31 36.54,21.22 arc-45 35.78,20.91 R3.2
  Bottom 0.406: RED.2 v40.16,28.73
N$5  (via drill 0.35)
  Top 0.406: v40.16,33.17 39.08,32.09 arc45 38.33,30.29 38.33,27.55 arc-45 37.52,25.58 36.92,24.99 arc45 36.66,24.34 36.66,24.19 arc-45 36.41,23.6 arc-45 35.49,23.22 R2.2
  Bottom 0.406: GREEN.2 v40.16,33.17
N$6  (via drill 0.35)
  Top 0.406: v40.13,37.64 40.13,36.74 arc-45 39.39,34.95 38.36,33.92 arc45 37.62,32.12 37.62,27.88 arc-45 36.85,26.03 arc-45 35.71,25.55 R1.2 34.72,25.5
  Bottom 0.406: BLUE.2 v40.13,37.64
N$7
  Bottom 0.406: Q1.2 36.98,31.72 | 36.98,31.72 arc75 38.89,33.17 arc-41 BLUE.1 | 36.98,31.72 37.45,31.25 arc45 39.25,30.51 GREEN.1 | RED.1 39.42,26.29 arc-56 38.26,27.46 arc-1 36.98,31.72
N$8
  Top 0.406: 51.57,22.5 arc45 R8.2 arc-45 51.35,22.48 52.49,22.01 53.12,21.39 arc-45 53.5,20.48 arc-45 53.35,20.13 IR12.VS
N$9
  Top 0.406: R11.2 IR1.VS
N$10
  Top 0.406: IR8.VS arc45 11.11,14.68 11.53,14.68 arc45 R14.2
N$11
  Top 0.406: R17.2 IR2.VS
N$12
  Top 0.406: R20.2 IR3.VS
N$13
  Top 0.406: R23.2 IR11.VS
N$14
  Top 0.406: R26.2 25.58,53.67 arc-45 25.86,54.34 arc-45 IR4.VS
N$15
  Top 0.406: R29.2 IR5.VS
N$16
  Top 0.406: IR10.VS R32.2
N$17
  Top 0.406: R5.2 IR9.VS
N$18
  Top 0.406: R35.2 IR6.VS
N$19
  Top 0.406: R38.2 IR7.VS
N$20
  Top 0.406: 42.48,19.12 R9.2 42.36,19.04 arc45 44.16,18.29 44.57,18.29 arc-45 46.36,17.55 47.06,16.85 arc-45 47.3,16.28 arc-45 46.86,15.24 R10.2 | 47.09,15.47 R10.2 | R10.2 47.1,14.87 arc45 47.92,14.53 49.25,14.53 arc45 49.86,14.79 IR12.VO
N$21
  Top 0.406: IR9.VO R6.2 R7.2
N$22
  Top 0.406: R31.2 R30.2 IR5.VO
N$23
  Top 0.406: IR1.VO R12.2 R13.2
N$25
  Top 0.406: R15.2 14.18,24.42 13.83,24.07 arc45 13.36,23.87 12.09,22.61 arc-45 10.44,21.92 10.14,21.92 arc-45 9.44,22.21 R16.2 7.82,21.71 arc45 7.08,19.91 IR8.VO
N$26
  Top 0.406: IR4.VO 33.07,55 arc-45 33.89,54.66 34.01,54.54 arc-45 34.45,53.5 R28.2 33.98,51.98 arc45 33.1,51.61 32.96,51.48 arc45 32.69,50.83 32.69,49.14 arc45 32.97,48.47 arc-45 33.13,48.07 R27.2
N$27
  Top 0.406: IR2.VO R18.2 R19.2
N$29
  Top 0.406: IR11.VO R24.2 R25.2
N$30
  Top 0.406: IR3.VO R21.2 R22.2
N$32
  Top 0.406: R34.2 R33.2 IR10.VO
N$34
  Top 0.406: IR6.VO R36.2 R37.2
N$36
  Top 0.406: R40.2 R39.2 IR7.VO
(copper drawn outside any net)
  shapes: Bottom circle x1

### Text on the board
tNames: STELA | XLC-CAPTUR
